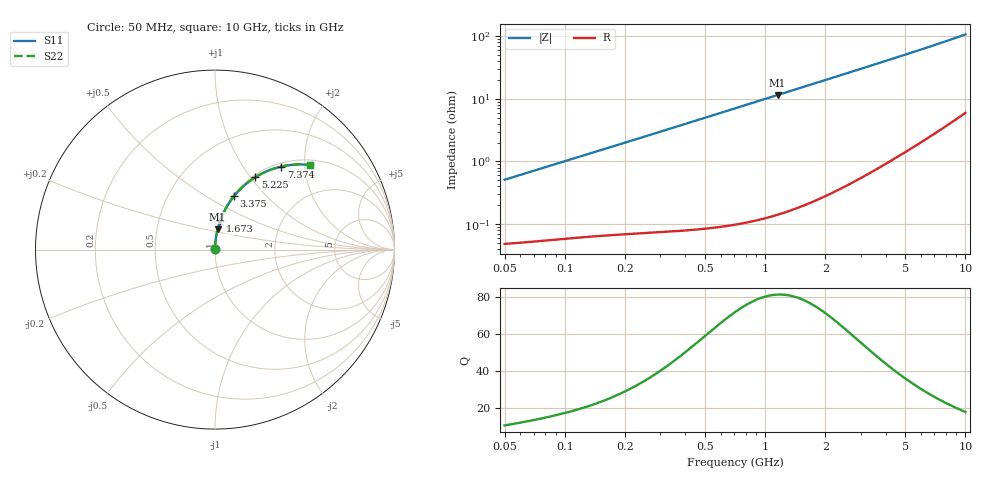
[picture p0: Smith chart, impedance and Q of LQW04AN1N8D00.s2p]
!Murata Part Number: LQW04AN1N8D00
!These Parameters are Measured in Series Mode Connection
!  o--[Z]--o
!Port1  Port2
!  o-------o
!Freq. Start=50[MHz] Stop=10[GHz], 401[Steps]
# Hz S RI R 50
!Freq.(Hz)	S 11(Real)	S 11(Imag)	S 21(Real)	S 21(Imag)	S 12(Real)	S 12(Imag)	S 22(Real)	S 22(Imag)
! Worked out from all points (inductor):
!   401 points, 50 MHz to 10 GHz, reference 50 ohm
!   read as one part in series: L = 1.61 nH near 51.34 MHz
!   highest Q = 81 at 1.154 GHz (marker M1), where L = 1.58 nH
!   S11 on the Smith chart (normalised r, x): 50 MHz: 1.00, +0.01; 1.673 GHz: 1.00, +0.33; 3.375 GHz: 1.01, +0.67; 5.225 GHz: 1.03, +1.05; 7.374 GHz: 1.06, +1.51; 10 GHz: 1.12, +2.11
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5e7  0.00051 0.00508  0.9995 -0.00508  0.9995 -0.00508  0.00051 0.00508
5.134228e7  0.000514 0.00522  0.9995 -0.00522  0.9995 -0.00522  0.000514 0.00522
1.214486e8  0.000764 0.0122  0.9992 -0.0122  0.9992 -0.0122  0.000764 0.0122
2.949953e8  0.0016 0.0293  0.9984 -0.0293  0.9984 -0.0293  0.0016 0.0293
4.689809e8  0.00298 0.0464  0.997 -0.0464  0.997 -0.0464  0.00298 0.0464
7.071068e8  0.00586 0.0697  0.9941 -0.0697  0.9941 -0.0697  0.00586 0.0697
9.094607e8  0.00919 0.0893  0.9908 -0.0893  0.9908 -0.0893  0.00919 0.0893
1.154331e9  0.0143 0.1127  0.9857 -0.1127  0.9857 -0.1127  0.0143 0.1127
1.67264e9  0.0288 0.1609  0.9712 -0.1609  0.9712 -0.1609  0.0288 0.1609
1.717543e9  0.0303 0.165  0.9697 -0.165  0.9697 -0.165  0.0303 0.165
2.095058e9  0.0442 0.1984  0.9558 -0.1984  0.9558 -0.1984  0.0442 0.1984
2.488741e9  0.061 0.2316  0.939 -0.2316  0.939 -0.2316  0.061 0.2316
2.917498e9  0.0819 0.2655  0.9181 -0.2655  0.9181 -0.2655  0.0819 0.2655
3.375117e9  0.1067 0.2989  0.8933 -0.2989  0.8933 -0.2989  0.1067 0.2989
4.171863e9  0.1546 0.3499  0.8454 -0.3499  0.8454 -0.3499  0.1546 0.3499
4.700058e9  0.1888 0.3784  0.8112 -0.3784  0.8112 -0.3784  0.1888 0.3784
5.225452e9  0.2239 0.4026  0.7761 -0.4026  0.7761 -0.4026  0.2239 0.4026
6.207365e9  0.2909 0.4374  0.7091 -0.4374  0.7091 -0.4374  0.2909 0.4374
7.37379e9  0.3693 0.4627  0.6307 -0.4627  0.6307 -0.4627  0.3693 0.4627
8.644138e9  0.4495 0.474  0.5505 -0.474  0.5505 -0.474  0.4495 0.474
9.738562e9  0.5125 0.4733  0.4875 -0.4733  0.4875 -0.4733  0.5125 0.4733
1e10  0.5267 0.4719  0.4733 -0.4719  0.4733 -0.4719  0.5267 0.4719
